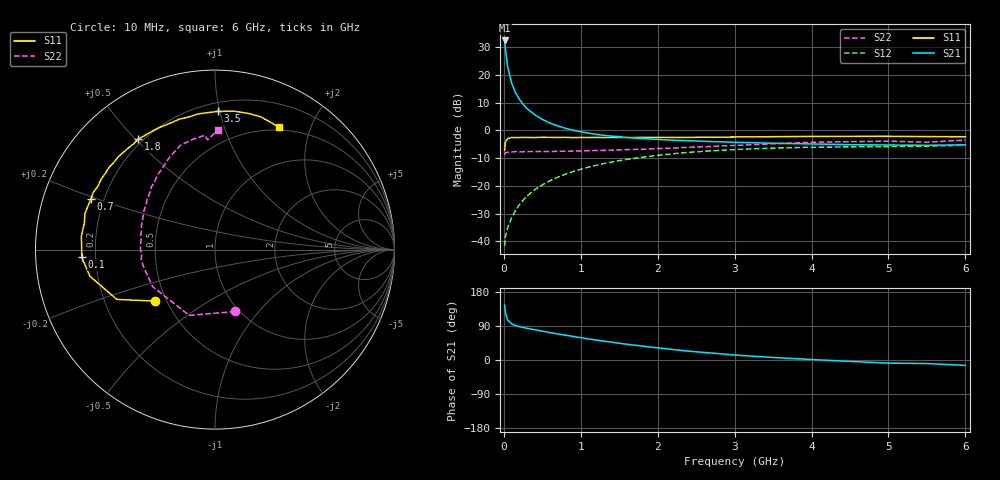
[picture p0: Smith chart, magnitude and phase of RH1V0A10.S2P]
! SIEMENS Small Signal Semiconductors
! BFR106
! Si NPN RF Bipolar Junction Transistor in SOT23
! VCE = 1 V  IC = 100 mA
! Common Emitter S-Parameters:  August  1996
# GHz  S  MA  R  50
!  f  S11  S21  S12  S22
! GHz  MAG  ANG  MAG  ANG  MAG  ANG  MAG  ANG
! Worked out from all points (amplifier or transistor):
!   36 points, 10 MHz to 6 GHz, reference 50 ohm
!   highest |S21| = 32.4 dB at 10 MHz (marker M1)
!   |S21| within 3 dB of that: start of sweep to 20.04 MHz
!   unconditionally stable (mu >= 1): start of sweep to 14 MHz; 37.98 MHz to end of sweep
!   at 250 MHz: K = 1.49, MAG = 13.1 dB, |S12| = -25.2 dB
!   at 1.4 GHz: K = 1.27, MAG = 1.6 dB, |S12| = -11.4 dB
!   at 6 GHz: K = 1.04, MAG = -1.2 dB, |S12| = -5.3 dB
!   S11 on the Smith chart (normalised r, x): 10 MHz: 0.43, -0.31; 100 MHz: 0.15, -0.03; 700 MHz: 0.15, +0.19; 1.8 GHz: 0.18, +0.51; 3.5 GHz: 0.26, +0.98; 6 GHz: 0.47, +1.55
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0.01  0.4393 -139.2  41.75 145.0  0.0082 56.4  0.3625 -72.0
0.02  0.6133 -153.1  29.58 125.5  0.012 48.6  0.3936 -111.4
0.05  0.7126 -168.0  13.89 105.2  0.0178 50.9  0.4045 -149.4
0.1  0.7442 -176.8  7.204 95.6  0.0264 59.9  0.4087 -166.2
0.15  0.743 179.4  4.843 91.2  0.0356 65.0  0.4155 -171.9
0.2  0.7446 176.9  3.681 88.1  0.0455 68.6  0.41 -175.6
0.25  0.7484 174.5  2.953 85.7  0.0552 69.6  0.413 -178.5
0.3  0.746 172.7  2.486 83.9  0.0655 70.9  0.4147 -180.0
0.4  0.7431 168.2  1.922 79.9  0.0851 71.0  0.4155 176.7
0.5  0.7518 164.8  1.582 76.3  0.1045 70.3  0.4157 173.9
0.6  0.7486 161.3  1.355 72.4  0.124 69.0  0.4158 171.8
0.7  0.7469 157.6  1.206 68.7  0.1435 67.6  0.4201 169.8
0.9  0.7422 151.6  1.009 62.2  0.1813 64.0  0.4237 165.1
1.1  0.7443 145.0  0.893 55.6  0.2175 60.3  0.4314 161.6
1.3  0.7439 138.8  0.814 49.6  0.2523 56.2  0.437 157.1
1.8  0.7505 124.9  0.715 36.9  0.3282 46.2  0.4565 147.3
2.2  0.7475 114.9  0.666 27.6  0.3797 38.4  0.48 139.4
3.5  0.7703 88.9  0.587 6.7  0.4802 16.2  0.5736 116.2
4.5  0.7815 76.0  0.553 -3.7  0.5046 2.9  0.6271 101.3
5  0.7824 70.9  0.546 -8.2  0.5115 -2.3  0.6396 95.1
5.5  0.7735 66.0  0.539 -9.3  0.5205 -4.6  0.6129 93.9
6  0.7685 62.4  0.55 -14.2  0.5402 -10.8  0.6682 88.4
